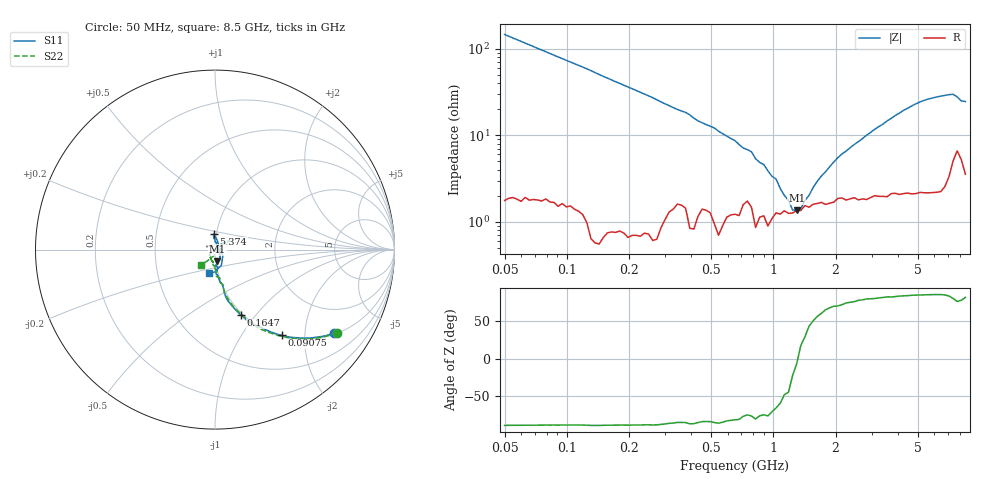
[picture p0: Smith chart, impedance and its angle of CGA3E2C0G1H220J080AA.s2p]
! S-parameter Generated by TDK Corporation
! Copyright(C) 2015 TDK Corporation.
! All Rights Reserved.
! TDK P/N: CGA3E2C0G1H220J080AA (Multilayer Ceramic Chip Capacitors)
! Property: C=22pF
! Size(LxWxT): 1.6x0.8x0.8mm, 0.063x0.031x0.031inches
! Model Type: s2p (Touchstone File Format Version 1.0)
! Frequency: DC=Yes Start=50MHz Stop=8500MHz 114points Log-sweep
! Note:
! Model Generated on Jun. 23, 2015
! Hash(MD5):
! Port Assignments:
!  1 ---| |--- 2
! Applicable Conditions:
!  Temperature = 25 degC
!  DC Bias Voltage = 0 V
!  Small Signal Operation
! Terms and conditions regarding TDK Simulation Models
! (1)This simulation model is being provided solely for informational purposes. Please refer to the specifications of the products in terms of detailed characteristics of such products.
! (2)In no event shall TDK Corporation of any of its subsidiaries be liable for any loss or damage arising, directly or indirectly,
!  From any information contained in this simulation model, including, but not limited to loss or damages arising from any inaccuracies, omissions or errors in connection with such information.
! (3)Any and all copyrights on this simulation model are owned by TDK Corporation.
!  Duplication or redistribution of this simulation model without prior written permission from TDK Corporation is prohibited.
! (4)This simulation model is subject to any modification or change without any prior notice.
! (5)Neither TDK Corporation nor any of its subsidiaries shall make any warranty, express or implied,
!  Including but not limited to the correctness, implied warranties of merchantability and fitness for a particular purpose with respect to this simulation models.
! (6)The use of this simulation model shall be deemed to have consented to the terms and conditions hereof.
# MHz S MA R 50
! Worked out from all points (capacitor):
!   113 points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, 50 MHz to 8.5 GHz, reference 50 ohm
!   read as one part in series: C = 21.8 pF near 50 MHz
!   lowest |Z| = 1.36 ohm at 1.297 GHz (marker M1)
!   series resonance near 1.314 GHz, so ESL is about 670 pH
!   S11 on the Smith chart (normalised r, x): 50 MHz: 1.04, -2.82; 90.75 MHz: 1.02, -1.53; 164.7 MHz: 0.98, -0.85; 5.374 GHz: 0.97, +0.17; 8.5 GHz: 0.90, -0.24
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50  0.8102 -35.1  0.5596 54.7  0.5603 54.7  0.8239 -34.3
90.75308  0.6052 -52.1  0.7627 37.9  0.7623 37.9  0.6301 -50.9
119.495  0.5054 -59.3  0.8332 30.7  0.8333 30.7  0.5283 -58.6
164.7224  0.3931 -68.4  0.8976 22.7  0.8972 22.8  0.4081 -66.7
285.5811  0.252 -77.5  0.9508 12.6  0.9509 12.7  0.2404 -77.8
651.9202  0.1206 -85.1  0.9695 3.0  0.9685 3.0  0.1115 -89.1
1296.926  0.06728 -78.5  0.9712 -3.6  0.9718 -3.6  0.06556 -108.4
1558.024  0.06177 -69.9  0.9701 -5.4  0.9703 -5.4  0.05667 -115.6
2147.718  0.05117 -54.5  0.9685 -8.8  0.9684 -8.8  0.04278 -129.4
2827.91  0.02899 -33.3  0.9673 -12.4  0.9677 -12.3  0.02934 -141.6
3099.524  0.02303 -7.4  0.965 -13.7  0.9651 -13.7  0.01696 -148.0
3244.963  0.01541 7.7  0.9651 -14.4  0.9634 -14.4  0.007963 -157.4
3397.226  0.018 24.2  0.9663 -15.2  0.966 -15.2  0.002955 -152.6
3556.634  0.02232 63.3  0.9639 -16.0  0.9646 -15.9  0.009816 48.2
3723.522  0.02618 69.1  0.9639 -16.8  0.9624 -16.8  0.01933 37.9
4272.658  0.05767 91.2  0.9596 -19.5  0.9607 -19.5  0.05514 36.2
5373.679  0.08725 94.9  0.9543 -24.9  0.956 -24.8  0.09539 30.5
6166.175  0.06735 86.4  0.9529 -28.8  0.9527 -28.7  0.07786 33.0
7075.547  0.03086 7.2  0.9402 -33.6  0.9402 -33.5  0.03715 47.3
7407.553  0.05534 -37.9  0.924 -35.1  0.9238 -35.2  0.01916 24.8
8119.031  0.1246 -90.7  0.9152 -35.9  0.9162 -35.8  0.0814 -125.5
8500  0.137 -104.5  0.9309 -37.6  0.9322 -37.5  0.1167 -133.0
